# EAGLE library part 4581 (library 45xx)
4-bit ALU
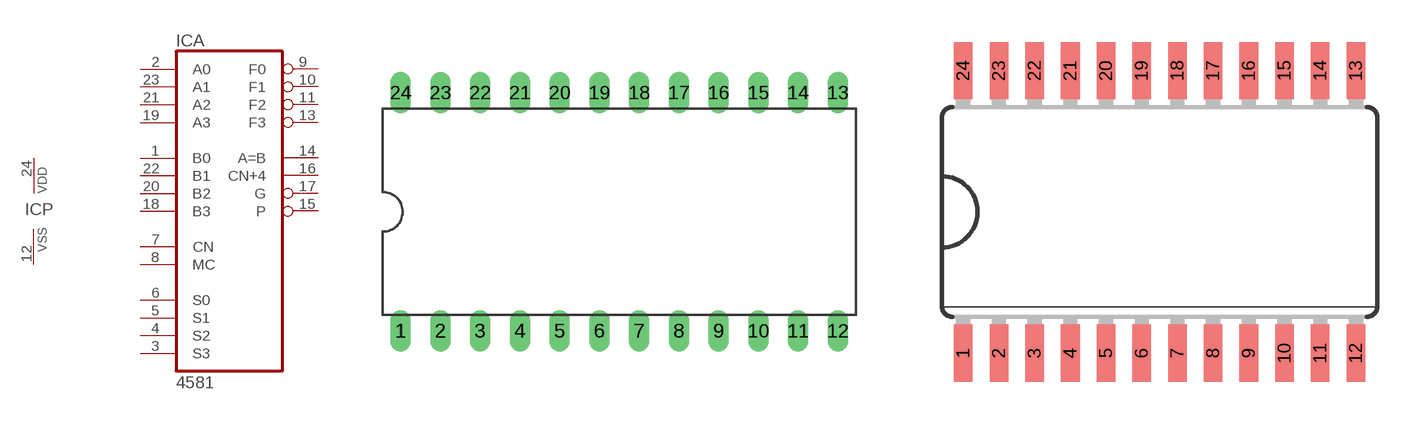
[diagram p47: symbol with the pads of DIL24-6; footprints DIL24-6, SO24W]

Designator prefix IC; gates A=4581 P=PWRN

## 4581N  [DIL24-6]
1  A:B0  in
2  A:A0  in
3  A:S3  in
4  A:S2  in
5  A:S1  in
6  A:S0  in
7  A:CN  in
8  A:MC  in
9  A:F0  out
10  A:F1  out
11  A:F2  out
12  P:VSS  pwr
13  A:F3  out
14  A:A=B  out
15  A:P  out
16  A:CN+4  out
17  A:G  out
18  A:B3  in
19  A:A3  in
20  A:B2  in
21  A:A2  in
22  A:B1  in
23  A:A1  in
24  P:VDD  pwr

## 4581D  [SO24W]
Pads as for DIL24-6

## Footprint DIL24-6 (pad centres in mm)
Dual In Line Package 0.6 inch
drill 0.813 long: 1 -13.97,-7.62; 2 -11.43,-7.62; 3 -8.89,-7.62; 4 -6.35,-7.62; 5 -3.81,-7.62; 6 -1.27,-7.62; 7 1.27,-7.62; 8 3.81,-7.62; 9 6.35,-7.62; 10 8.89,-7.62; 11 11.43,-7.62; 12 13.97,-7.62; 13 13.97,7.62; 14 11.43,7.62; 15 8.89,7.62; 16 6.35,7.62; 17 3.81,7.62; 18 1.27,7.62; 19 -1.27,7.62; 20 -3.81,7.62; 21 -6.35,7.62; 22 -8.89,7.62; 23 -11.43,7.62; 24 -13.97,7.62

## Footprint SO24W (pad centres in mm)
Wide Small Outline package 300 mil
smd 0.66 x 2.032: 1 -6.985,-5.029; 2 -5.715,-5.029; 3 -4.445,-5.029; 4 -3.175,-5.029; 5 -1.905,-5.029; 6 -0.635,-5.029; 7 0.635,-5.029; 8 1.905,-5.029; 9 3.175,-5.029; 10 4.445,-5.029; 11 5.715,-5.029; 12 6.985,-5.029; 13 6.985,5.029; 14 5.715,5.029; 15 4.445,5.029; 16 3.175,5.029; 17 1.905,5.029; 18 0.635,5.029; 19 -0.635,5.029; 20 -1.905,5.029; 21 -3.175,5.029; 22 -4.445,5.029; 23 -5.715,5.029; 24 -6.985,5.029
